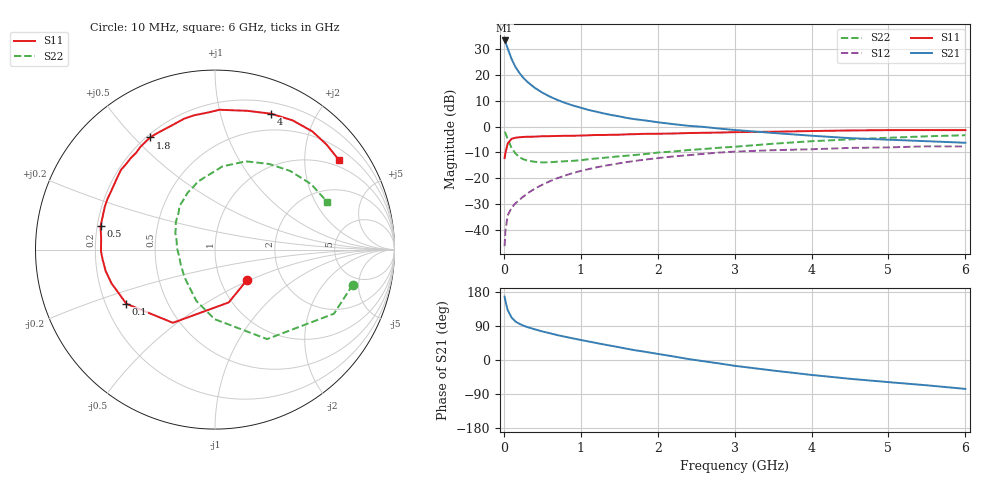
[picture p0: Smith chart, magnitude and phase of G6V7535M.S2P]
! SIEMENS Small Signal Semiconductors
! BFG193
! Si NPN RF Bipolar Junction Transistor in SOT223
! VCE = 0.75 V  IC = 35 mA
! Common Emitter S-Parameters:  August  1996
# GHz  S  MA  R  50
!  f  S11  S21  S12  S22
! GHz  MAG  ANG  MAG  ANG  MAG  ANG  MAG  ANG
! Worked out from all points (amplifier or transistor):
!   36 points, 10 MHz to 6 GHz, reference 50 ohm
!   highest |S21| = 33.2 dB at 10 MHz (marker M1)
!   |S21| within 3 dB of that: start of sweep to 49.03 MHz
!   unconditionally stable (mu >= 1): 317.6 MHz to end of sweep
!   at 250 MHz: K = 0.95, MSG = 23.0 dB, |S12| = -27.1 dB
!   at 1.4 GHz: K = 1.11, MAG = 7.5 dB, |S12| = -14.7 dB
!   at 6 GHz: K = 1.02, MAG = -0.2 dB, |S12| = -7.7 dB
!   S11 on the Smith chart (normalised r, x): 10 MHz: 1.33, -0.48; 100 MHz: 0.29, -0.26; 500 MHz: 0.21, +0.10; 1.8 GHz: 0.21, +0.56; 4 GHz: 0.31, +1.45; 6 GHz: 0.80, +2.91
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0.01  0.2462 -43.8  45.94 167.4  0.0049 80.5  0.7919 -14.3
0.02  0.3041 -75.4  43.15 156.6  0.0095 71.9  0.7529 -28.3
0.05  0.4705 -119.9  32.22 131.7  0.0192 57.3  0.5769 -59.8
0.1  0.5789 -148.6  20.29 112.3  0.027 52.9  0.3873 -90.4
0.15  0.6069 -162.1  14.21 101.7  0.0327 53.5  0.3037 -110.1
0.2  0.621 -169.1  10.97 95.7  0.0381 56.1  0.2577 -122.5
0.25  0.6287 -175.0  8.841 91.0  0.044 57.5  0.2342 -134.2
0.3  0.6353 -179.2  7.424 87.2  0.0505 59.4  0.222 -142.1
0.4  0.6375 174.3  5.62 81.2  0.0628 60.5  0.2087 -156.1
0.5  0.6508 168.5  4.515 75.5  0.0753 60.3  0.2033 -165.9
0.6  0.6524 163.6  3.78 70.5  0.0882 59.7  0.2044 -173.1
0.7  0.6588 158.9  3.248 65.5  0.1012 58.3  0.2095 -179.6
0.9  0.6639 150.7  2.545 57.0  0.1268 54.7  0.2176 168.6
1.1  0.6777 143.1  2.095 48.9  0.1504 50.8  0.2335 160.2
1.4  0.6933 132.5  1.668 37.4  0.1839 43.8  0.2577 148.0
1.8  0.722 120.1  1.333 22.9  0.2265 34.4  0.2903 134.2
2.2  0.7336 108.6  1.115 9.6  0.2642 24.2  0.329 122.1
3.5  0.7939 76.9  0.752 -27.8  0.3495 -8.6  0.4657 84.8
4  0.8189 67.6  0.665 -39.4  0.3645 -18.1  0.521 70.7
4.5  0.8399 59.0  0.597 -49.6  0.3867 -27.8  0.565 57.6
5.5  0.8537 43.1  0.521 -66.8  0.415 -49.8  0.6483 34.2
6  0.8524 35.7  0.486 -76.3  0.4129 -62.3  0.6791 23.0
